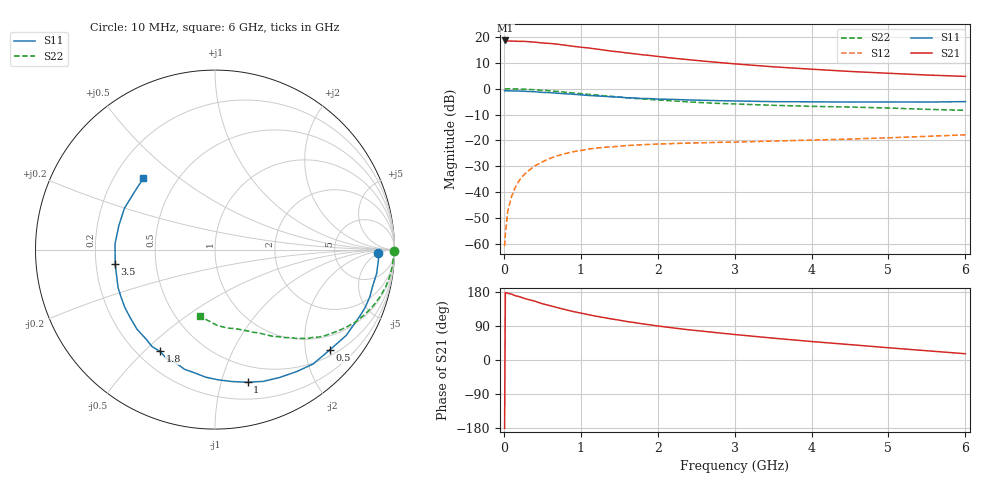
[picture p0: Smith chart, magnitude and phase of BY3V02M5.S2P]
! SIEMENS Small Signal Semiconductors
! BFY420
! Si NPN RF SIEGET Grounded Emitter Transistor in MICRO-X
! VCE = 3 V  IC = 2.5 mA
! Common Emitter S-Parameters:  October  1996
# GHz  S  MA  R  50
!  f  S11  S21  S12  S22
! GHz  MAG  ANG  MAG  ANG  MAG  ANG  MAG  ANG
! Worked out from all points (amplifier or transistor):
!   36 points, 10 MHz to 6 GHz, reference 50 ohm
!   highest |S21| = 18.7 dB at 20 MHz (marker M1)
!   |S21| within 3 dB of that: start of sweep to 1.124 GHz
!   unconditionally stable (mu >= 1): 3.823 GHz to end of sweep
!   at 250 MHz: K = 0.07, MSG = 26.0 dB, |S12| = -33.7 dB
!   at 1.4 GHz: K = 0.33, MSG = 18.5 dB, |S12| = -22.5 dB
!   at 6 GHz: K = 1.21, MAG = 8.5 dB, |S12| = -17.9 dB
!   S11 on the Smith chart (normalised r, x): 10 MHz: 20, -4; 500 MHz: 0.63, -2.53; 1 GHz: 0.35, -1.22; 1.8 GHz: 0.29, -0.56; 3.5 GHz: 0.28, -0.07; 6 GHz: 0.32, +0.38
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0.01  0.9097 -1.2  8.54 -179.9  0.0009 88.6  0.9957 -0.5
0.02  0.9136 -1.9  8.578 178.2  0.0015 85.9  0.9896 -0.8
0.05  0.9118 -4.2  8.351 176.1  0.0042 83.7  0.9962 -2.0
0.1  0.9104 -8.5  8.343 173.9  0.0082 85.9  0.9934 -4.2
0.15  0.902 -12.6  8.289 169.6  0.0125 81.3  0.9898 -6.3
0.2  0.902 -16.9  8.257 167.3  0.0167 81.2  0.986 -8.2
0.3  0.8872 -25.0  8.172 160.6  0.0245 75.9  0.9732 -12.4
0.4  0.8735 -33.2  7.955 155.3  0.032 70.9  0.955 -16.2
0.5  0.8494 -41.1  7.679 148.5  0.0384 67.2  0.9337 -19.9
0.7  0.8183 -56.1  7.249 138.1  0.0507 59.5  0.8843 -26.8
0.8  0.7977 -63.4  6.934 132.8  0.0556 55.4  0.8567 -29.8
1  0.7611 -76.2  6.358 123.8  0.0637 49.5  0.8043 -35.2
1.1  0.741 -82.7  6.143 119.6  0.0679 46.8  0.7802 -37.8
1.4  0.6963 -99.3  5.326 108.4  0.075 39.9  0.7117 -44.1
1.6  0.667 -109.5  4.919 101.5  0.0794 36.4  0.6683 -47.7
1.8  0.6445 -118.5  4.539 95.5  0.0825 33.4  0.6348 -50.6
2.2  0.621 -134.4  3.895 84.7  0.0869 28.7  0.5814 -56.2
2.8  0.5866 -153.1  3.215 71.4  0.0916 24.8  0.5188 -63.1
3.5  0.5622 -171.6  2.654 57.7  0.097 22.2  0.4778 -70.1
4.5  0.5522 165.8  2.158 40.6  0.1062 20.1  0.4421 -81.1
5.5  0.5516 144.8  1.839 24.4  0.1199 18.2  0.3994 -94.9
6  0.5633 135.2  1.731 16.5  0.128 16.9  0.3818 -102.9
